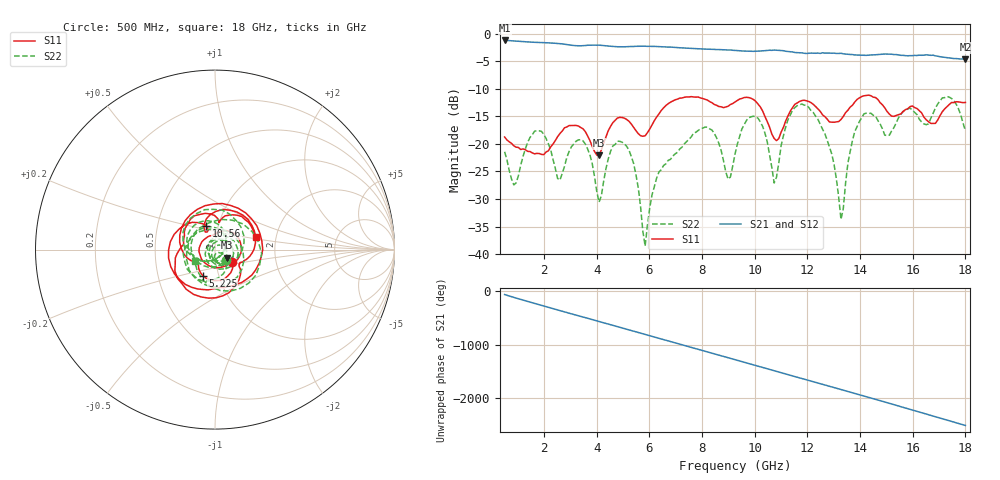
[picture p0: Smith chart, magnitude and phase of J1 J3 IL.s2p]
!Agilent Technologies,N5230A,MY45001360,A.07.50.67
!Agilent N5230A: A.07.50.67
!Date: Tuesday, April 16, 2024 17:34:58
!Correction: S11(Full 2 Port(1,2))
!S21(Full 2 Port(1,2))
!S12(Full 2 Port(1,2))
!S22(Full 2 Port(1,2))
!S2P File: Measurements: S11, S21, S12, S22:
# Hz S  dB  R 50
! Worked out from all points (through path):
!   201 points, 500 MHz to 18 GHz, reference 50 ohm
!   highest |S21| = -1.25 dB at 500 MHz (marker M1); lowest = -4.6 dB at 18 GHz (marker M2)
!   group delay of S21, straight-line fit = 387 ps
!   lowest |S11| = -22.1 dB at 4.088 GHz (marker M3), VSWR 1.17, Z = 56.7 - j5.13 ohm
!   |S11| at or under -10 dB: start of sweep to end of sweep
!   |S22| runs from -38.5 to -11.4 dB; largest |S21 - S12| = 0.008
!   S11 on the Smith chart (normalised r, x): 500 MHz: 1.19, -0.17; 5.225 GHz: 0.84, -0.25; 10.56 GHz: 0.88, +0.24; 18 GHz: 1.57, +0.23
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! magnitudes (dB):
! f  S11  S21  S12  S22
! 500 MHz  -18.8  -1.3  -1.2  -21.4
! 850 MHz  -20.3  -1.3  -1.3  -27.4
! 1.9 GHz  -21.9  -1.6  -1.6  -17.7
! 2.6 GHz  -18.1  -1.8  -1.8  -26.6
! 3.475 GHz  -17.3  -2.2  -2.2  -19.4
! 4.088 GHz  -22.1  -2.1  -2.1  -30.6
! 4.612 GHz  -16.1  -2.3  -2.3  -20.4
! 5.225 GHz  -15.9  -2.4  -2.4  -21.2
! 5.838 GHz  -18.5  -2.3  -2.3  -38.5
! 6.362 GHz  -14.6  -2.4  -2.4  -25.1
! 8.113 GHz  -11.9  -2.8  -2.8  -17.0
! 9.25 GHz  -12.4  -3.1  -3.1  -21.9
! 9.95 GHz  -12.0  -3.2  -3.2  -15.0
! 10.56 GHz  -17.0  -3.0  -3.0  -22.0
! 10.74 GHz  -19.0  -3.0  -3.1  -27.1
! 11.44 GHz  -13.4  -3.3  -3.4  -13.9
! 12.22 GHz  -12.8  -3.6  -3.5  -14.3
! 13.28 GHz  -15.6  -3.6  -3.7  -33.7
! 13.97 GHz  -11.7  -3.9  -3.9  -15.9
! 15.11 GHz  -14.6  -3.7  -3.7  -18.4
! 17.3 GHz  -13.3  -4.4  -4.4  -11.4
! 18 GHz  -12.5  -4.6  -4.7  -17.6
